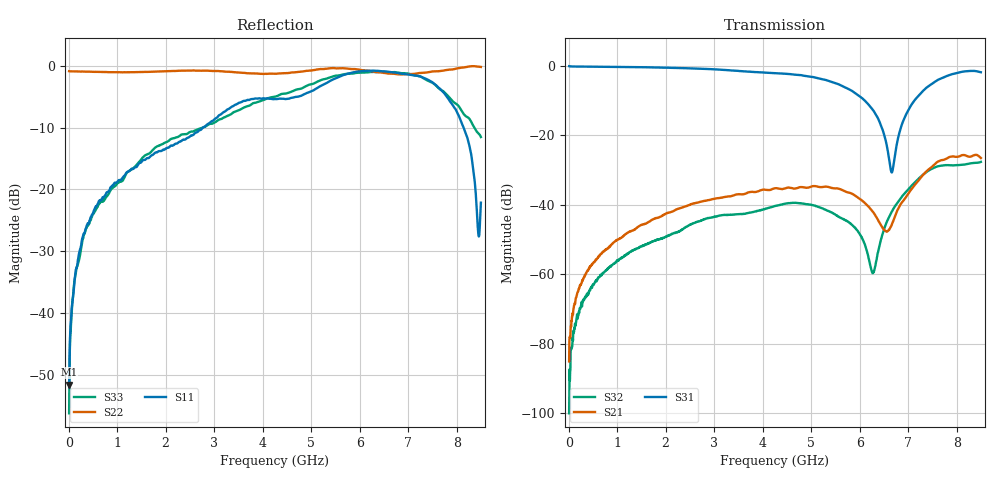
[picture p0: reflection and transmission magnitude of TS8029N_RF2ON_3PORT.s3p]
!Created with skrf (http://scikit-rf.org).
# GHz S RI R 50.0
!freq ReS11 ImS11 ReS12 ImS12 ReS13 ImS13
! ReS21 ImS21 ReS22 ImS22 ReS23 ImS23
! ReS31 ImS31 ReS32 ImS32 ReS33 ImS33
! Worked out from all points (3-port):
!   1601 points, 10 MHz to 8.5 GHz, reference 50 ohm
!   strongest paths, dB at 10 MHz, 2.132 GHz, 4.255 GHz, 6.378 GHz, 8.5 GHz:
!     S31: 0.0, -0.5, -2.0, -15.1, -1.8
!     S21: -85.1, -42.0, -35.2, -44.3, -26.5
!     S32: -100.1, -48.4, -40.3, -53.7, -27.6
!   lowest |S11| = -51.6 dB at 10 MHz (marker M1), VSWR 1.01, Z = 50 + j0.263 ohm
!   |S11| at or under -10 dB: start of sweep to 2.768 GHz; 8.144 GHz to end of sweep
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0.01  0.000245 0.00263  2.56e-05 6.93e-05  0.9948 -0.00804
      2.66e-05 4.88e-05  -0.9051 0.00342  2.44e-05 1.19e-05
      0.9949 -0.00806  9.14e-06 3.89e-06  0.00145 0.00052
0.1426563  0.00891 -0.0194  7.19e-05 0.000449  0.9814 -0.0545
           9.7e-05 0.000422  -0.9011 0.0341  2.94e-05 -0.000198
           0.9813 -0.0546  7.08e-05 -0.00018  0.00667 -0.0197
0.625525  -0.00258 -0.0802  -0.000129 0.00181  0.9503 -0.2236
          -0.000117 0.00182  -0.879 0.1552  -0.000549 -0.00075
          0.9502 -0.2236  -0.000541 -0.000731  -0.0124 -0.0747
4.255  -0.5379 0.0311  0.00892 0.015  -0.077 -0.7887
       0.00886 0.0149  -0.3156 0.8031  -0.000228 0.0096
       -0.0777 -0.7869  -0.000196 0.00965  -0.5621 -0.0123
5.761975  -0.5181 0.6925  0.0131 0.0075  -0.3455 -0.3174
          0.0131 0.0075  -0.014 0.9481  0.00404 0.00405
          -0.3453 -0.3171  0.00404 0.00405  -0.5786 0.6412
6.271375  -0.2264 0.8859  0.00708 0.00371  -0.2131 -0.0968
          0.00707 0.00369  0.0275 0.9021  -0.000242 0.001
          -0.2131 -0.0968  -0.000251 0.001  -0.3767 0.8099
6.664038  0.0205 0.8869  -0.00134 0.00507  -0.000767 -0.0293
          -0.00137 0.00505  0.1503 0.8504  -0.00762 0.00238
          -0.000865 -0.0293  -0.00765 0.0024  0.0619 0.8855
7.263644  0.4861 0.6552  -0.00946 0.023  0.2829 -0.2935
          -0.0095 0.0229  0.4042 0.7787  -0.0145 0.0211
          0.2828 -0.2921  -0.0145 0.0211  0.5576 0.5947
8.043662  0.3941 0.0271  0.0206 0.0452  0.0158 -0.8036
          0.0206 0.0452  0.5779 0.7642  0.0124 0.0353
          0.0156 -0.8045  0.0124 0.0353  0.4272 0.1986
8.5  -0.0247 0.0741  0.0301 0.0364  -0.2283 -0.7805
     0.0301 0.0364  0.527 0.8254  0.0152 0.0388
     -0.228 -0.7807  0.0151 0.0388  0.2635 -0.0322
